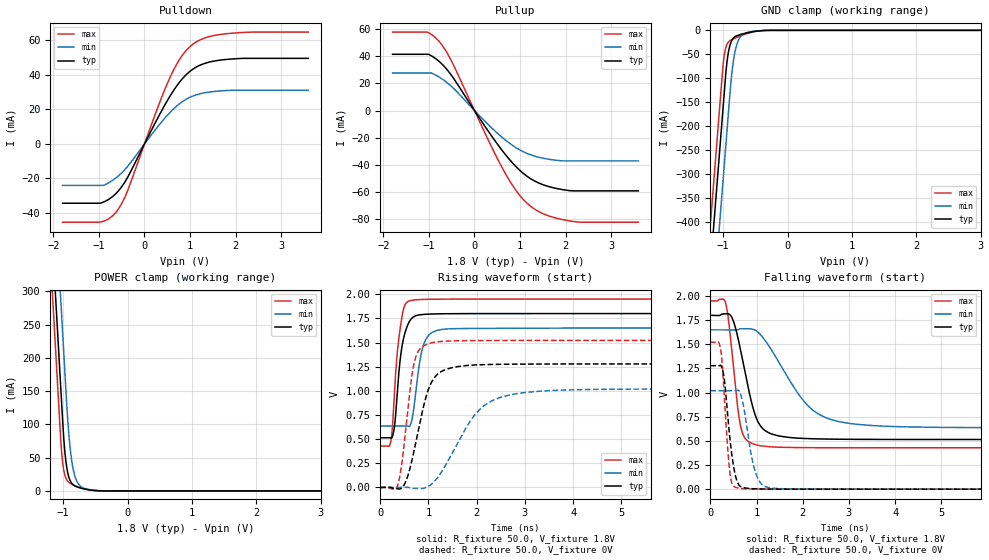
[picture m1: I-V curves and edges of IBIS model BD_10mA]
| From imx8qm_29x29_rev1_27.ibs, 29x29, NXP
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[Model] BD_10mA
Model_type I/O
Polarity   Non-Inverting
Enable   Active-Low
| C_comp min and max val. don't necessarily correlate with the min and max pvt
| but are the smallest and greatest pad capacitance found.
| var   typ   min   max
C_comp   1.59190pF  1.51745pF  1.65990pF
Vinl = 577.5mV
Vinh = 1.2675V
Vmeas = 900.0mV   | Reference voltage for timing measurements
Cref  = 15.0pF   | Timing specification test load capacitance value
Rref  = 1.0MOhm   | Timing specification test load resistance value
Vref  = 1.8V   | Timing specification test load voltage
[Model Spec]
| :
Vinl 630.00000mV 577.50000mV 682.50000mV
Vinh 1.17000V 1.07250V 1.26750V
| variable   typ   min   max
[Temperature Range] 25.0 125.0 -40.0
| variable   typ   min   max
[Voltage Range] 1.8V 1.65V 1.95V
| variable   typ   min   max
[POWER Clamp Reference] 1.8V 1.65V 1.95V
| variable   typ   min   max
[GND Clamp Reference] 0V 0V 0V
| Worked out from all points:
|   slope of the pulldown table from 0 to 0.27 V, typ, clamps not added: 19.4 ohm
|   slope of the pullup table from 0 to 0.27 V, typ, clamps not added: 19.9 ohm
|   GND clamp passes 1 mA (typ) near -0.44 V on its own axis
|   POWER clamp passes 1 mA (typ) near -0.55 V on its own axis
|   rising waveform, R_fixture 50.0, V_fixture 1.8V: 20-80 % time 161ps typ, 179ps min, 146ps max; typ from 0.515 V to 1.8 V
|   falling waveform, R_fixture 50.0, V_fixture 1.8V: 20-80 % time 360ps typ, 853ps min, 205ps max; typ from 1.8 V to 0.515 V
|   rising waveform, R_fixture 50.0, V_fixture 0V: 20-80 % time 358ps typ, 757ps min, 214ps max; typ from 0 V to 1.28 V
|   falling waveform, R_fixture 50.0, V_fixture 0V: 20-80 % time 167ps typ, 222ps min, 126ps max; typ from 1.28 V to 0 V
[POWER Clamp]
-1.8V     1.452A     1.584A     1.373A
-1.18V    398.2mA    529.9mA    318.8mA
-1.15V    347.2mA    478.9mA    267.8mA
-1.12V    296.2mA    427.9mA    216.8mA
-1.04V    160.2mA    291.9mA    80.78mA
-1V       92.69mA    223.9mA    36.89mA
-950mV    39.12mA    138.9mA    17.72mA
-890mV    15.28mA    63.28mA    11.47mA
-820mV    7.619mA    23.03mA    8.072mA
-710mV    3.877mA    5.679mA    4.137mA
-440mV    198.6uA    468.9uA    81.6uA
3.6V      0A         0A         0A
[GND Clamp]
-1.8V     -1.52A     -1.672A    -1.429A
-1.21V    -517.1mA   -668.6mA   -425.9mA
-1.12V    -364.1mA   -515.6mA   -272.9mA
-1.04V    -228.1mA   -379.6mA   -136.9mA
-990mV    -143.1mA   -294.6mA   -59.11mA
-960mV    -92.41mA   -243.6mA   -36.73mA
-930mV    -55.69mA   -192.6mA   -26.66mA
-870mV    -22.37mA   -96.04mA   -19.77mA
-810mV    -12.81mA   -41.2mA    -16.04mA
-700mV    -7.565mA   -8.808mA   -10.1mA
-450mV    -1.118mA   -1.064mA   -1.253mA
3.6V      32.66uA    16.11uA    55.52uA
| variable   typ   min   max
[Pullup Reference] 1.8V 1.65V 1.95V
| variable   typ   min   max
[Pulldown Reference] 0V 0V 0V
[Pullup]
-1.8V     41.45mA    27.68mA    57.81mA
-1.04V    41.45mA    27.68mA    57.81mA
-950mV    40.39mA    27.68mA    56.16mA
-750mV    35.39mA    24.1mA     49.83mA
-450mV    23.29mA    16mA       32.79mA
310mV     -15.53mA   -10.57mA   -22.22mA
650mV     -31.2mA    -20.92mA   -44.7mA
990mV     -43.87mA   -28.88mA   -62.31mA
1.24V     -50.34mA   -32.69mA   -70.69mA
1.65V     -56.18mA   -35.96mA   -77.83mA
2.17V     -59.16mA   -37.08mA   -81.71mA
3.6V      -59.16mA   -37.08mA   -82.24mA
[Pulldown]
-1.8V     -34.33mA   -24mA      -45.32mA
-950mV    -34.16mA   -24mA      -45.08mA
-790mV    -32.16mA   -22.54mA   -43.44mA
-600mV    -27.97mA   -19.09mA   -38.63mA
-370mV    -19.3mA    -13.02mA   -26.96mA
310mV     15.95mA    10.63mA    22.4mA
570mV     28.11mA    18.52mA    39.07mA
820mV     37.42mA    24.3mA     50.97mA
1.07V     43.46mA    27.84mA    57.94mA
1.33V     46.73mA    29.68mA    61.45mA
1.8V      48.97mA    30.95mA    63.86mA
3.6V      49.59mA    31.11mA    64.81mA
[Ramp]
dV/dt_r 767.03797mV/358.46884ps 611.86389mV/757.03995ps 912.92019mV/214.02531ps
dV/dt_f 771.27832mV/359.59396ps 608.28171mV/852.91685ps 912.92618mV/205.15859ps
R_load = 50.0
| Removed startup time: 0s 0s 0s  .
| Removed end time: 20.0ns.
[Rising Waveform]
R_fixture   = 50.0
V_fixture   = 1.8V
V_fixture_min = 1.65V
V_fixture_max = 1.95V
0s        514.6mV    636.3mV    428.5mV
192ps     514.8mV    636.3mV    430.6mV
264ps     547.1mV    636.3mV    712.7mV
344ps     917.2mV    636.3mV    1.347V
444ps     1.44V      636.3mV    1.75V
672ps     1.759V     740.3mV    1.939V
812ps     1.786V     1.281V     1.945V
908ps     1.792V     1.491V     1.947V
1.336ns   1.798V     1.639V     1.949V
20ns      1.8V       1.65V      1.95V
| Removed startup time: 0s 0s 0s  .
| Removed end time: 20.0ns.
[Falling Waveform]
R_fixture   = 50.0
V_fixture   = 1.8V
V_fixture_min = 1.65V
V_fixture_max = 1.95V
0s        1.8V       1.65V      1.95V
320ps     1.816V     1.65V      1.944V
476ps     1.769V     1.65V      1.383V
600ps     1.564V     1.653V     818.6mV
688ps     1.363V     1.661V     592.8mV
920ps     849.1mV    1.657V     471mV
1.096ns   649mV      1.595V     449.1mV
2.148ns   522.8mV    848.6mV    429.6mV
3.136ns   516mV      673.6mV    428.5mV
20ns      514.5mV    636.2mV    428.5mV
| Removed startup time: 0s 0s 0s  .
| Removed end time: 20.0ns.
[Rising Waveform]
R_fixture   = 50.0
V_fixture   = 0V
V_fixture_min = 0V
V_fixture_max = 0V
0s        205.5nV    447.2nV    494nV
344ps     -14.7mV    453.9nV    2.142mV
512ps     42.67mV    -13.26uV   523.8mV
644ps     253mV      -8.023mV   1.113V
736ps     462.2mV    -10.67mV   1.35V
956ps     950.1mV    948.1uV    1.479V
1.136ns   1.145V     70.37mV    1.504V
2.072ns   1.27V      811.5mV    1.521V
3.076ns   1.277V     986.4mV    1.522V
20ns      1.278V     1.02V      1.522V
| Removed startup time: 0s 0s 0s  .
| Removed end time: 20.0ns.
[Falling Waveform]
R_fixture   = 50.0
V_fixture   = 0V
V_fixture_min = 0V
V_fixture_max = 0V
0s        1.278V     1.02V      1.521V
184ps     1.277V     1.02V      1.519V
272ps     1.222V     1.02V      1.206V
360ps     862.6mV    1.02V      531.1mV
432ps     490.2mV    1.02V      140.7mV
532ps     166.9mV    1.019V     22.28mV
632ps     35.97mV    1.009V     9.367mV
984ps     3.284mV    165.6mV    966.8uV
1.344ns   803.3uV    10.65mV    278.1uV
20ns      246.5nV    513nV      523.5nV
